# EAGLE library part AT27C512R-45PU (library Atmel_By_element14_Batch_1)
OTP EPROM
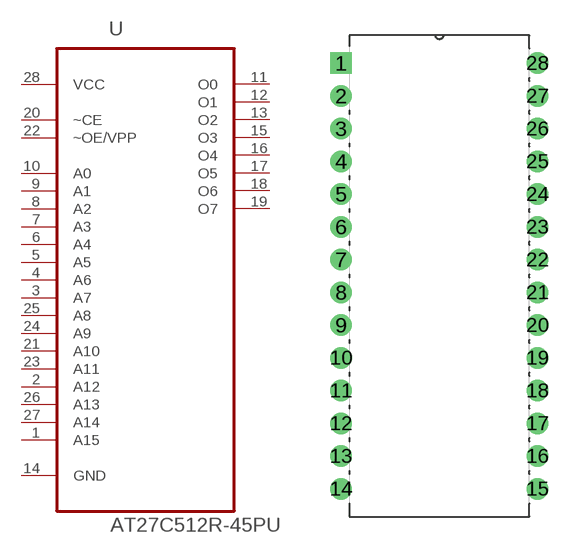
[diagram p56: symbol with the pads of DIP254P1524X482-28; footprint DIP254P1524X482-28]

Designator prefix U

## AT27C512R-45PU (DESCRIPTION: OTP EPROM; MPN: AT27C512R-45PU; OC_FARNELL: 1455028; OC_NEWARK: 58M3826; PACKAGE: PDIP-28; SUPPLIER: ATMEL)  [DIP254P1524X482-28]
1  A15  pwr
2  A12  in
3  A7  in
4  A6  in
5  A5  in
6  A4  in
7  A3  in
8  A2  in
9  A1  in
10  A0  in
11  O0  out
12  O1  out
13  O2  out
14  GND  pas
15  O3  out
16  O4  out
17  O5  out
18  O6  out
19  O7  out
20  ~CE  in
21  A10  in
22  ~OE/VPP  in
23  A11  in
24  A9  in
25  A8  in
26  A13  in
27  A14  in
28  VCC  pwr

## Footprint DIP254P1524X482-28 (pad centres in mm)
drill 1.118 square: 1 -15.24,33.02
drill 1.118: 2 -15.24,30.48; 3 -15.24,27.94; 4 -15.24,25.4; 5 -15.24,22.86; 6 -15.24,20.32; 7 -15.24,17.78; 8 -15.24,15.24; 9 -15.24,12.7; 10 -15.24,10.16; 11 -15.24,7.62; 12 -15.24,5.08; 13 -15.24,2.54; 14 -15.24,0; 15 0,0; 16 0,2.54; 17 0,5.08; 18 0,7.62; 19 0,10.16; 20 0,12.7; 21 0,15.24; 22 0,17.78; 23 0,20.32; 24 0,22.86; 25 0,25.4; 26 0,27.94; 27 0,30.48; 28 0,33.02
